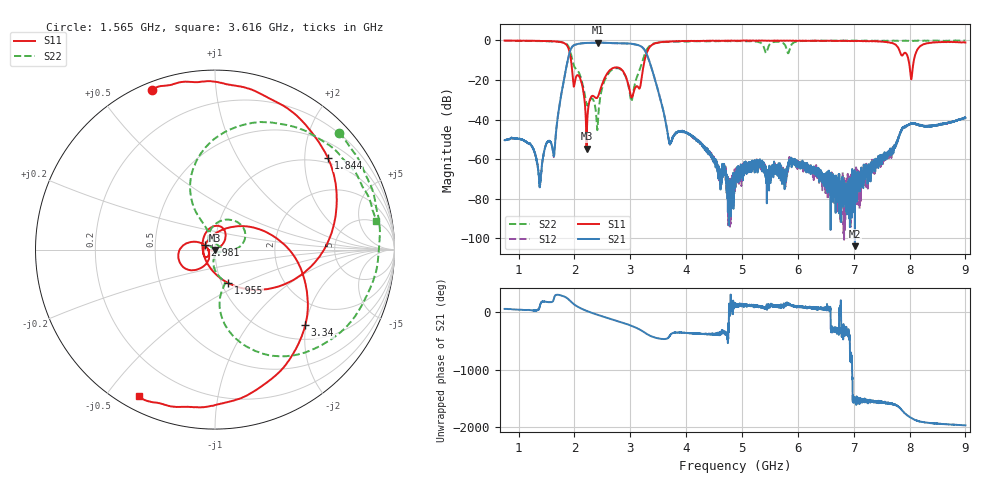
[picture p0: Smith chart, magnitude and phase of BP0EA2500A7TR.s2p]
!Agilent Technologies,E8358A,US41080443,A.07.50.56
!Agilent E8358A: A.07.50.56
!Date: Friday, November 20, 2015 10:47:14
!Correction: S11(Full 2 Port(1,2))
!S21(Full 2 Port(1,2))
!S12(Full 2 Port(1,2))
!S22(Full 2 Port(1,2))
!S2P File: Measurements: S11, S21, S12, S22:
# Hz S  dB  R 50
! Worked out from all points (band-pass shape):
!   6401 points, 750 MHz to 9 GHz, reference 50 ohm
!   highest |S21| = -1.11 dB at 2.414 GHz (marker M1); lowest = -104.0 dB at 7.021 GHz (marker M2)
!   |S21| within 3 dB of the highest: 1.94 GHz to 3.238 GHz (1.298 GHz wide, 50.1 % of centre)
!   lowest |S11| = -54.8 dB at 2.217 GHz (marker M3), VSWR 1.00, Z = 50 - j0.176 ohm
!   |S11| at or under -10 dB: 1.939 GHz to 3.257 GHz (1.319 GHz wide, 50.8 % of centre); 7.983 GHz to 8.077 GHz (94.32 MHz wide, 1.17 % of centre)
!   |S22| runs from -45.3 to 0.0 dB; largest |S21 - S12| = 0.0055
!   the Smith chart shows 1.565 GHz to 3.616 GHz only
!   S11 on the Smith chart (normalised r, x): 1.565 GHz: 0.03, +0.68; 1.844 GHz: 0.86, +2.56; 1.955 GHz: 1.07, -0.42; 2.981 GHz: 0.89, +0.04; 3.34 GHz: 1.34, -1.98; 3.616 GHz: 0.06, -0.61
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7.5e8  -0.05 161.1  -50.34 53.8  -50.43 54.1  -0.18 131.6
1.211484e9  -0.16 141.1  -52.47 32.4  -52.49 32.3  -0.30 90.8
1.377773e9  -0.23 129.8  -74.27 98.5  -71.71 86.6  -0.35 71.2
1.564688e9  -0.38 111.5  -51.08 170.0  -51.16 169.5  -0.44 43.3
1.64332e9  -0.46 99.7  -56.13 -92.6  -55.97 -93.4  -0.54 28.4
1.844414e9  -1.83 39.1  -14.98 -104.5  -15.02 -104.6  -1.44 -30.9
1.955273e9  -13.99 -68.5  -3.37 164.8  -3.40 164.8  -8.99 -85.0
2.12543e9  -21.07 48.6  -1.46 58.3  -1.50 58.3  -19.68 -92.1
2.216953e9  -54.76 -74.8  -1.25 19.6  -1.28 19.6  -32.11 -70.8
2.41418e9  -28.70 -148.7  -1.11 -48.8  -1.14 -48.8  -44.56 -152.6
2.665547e9  -14.32 -145.5  -1.31 -125.1  -1.34 -125.0  -14.96 69.1
2.981367e9  -24.19 157.0  -1.58 135.7  -1.61 135.7  -24.98 2.0
3.206953e9  -18.30 67.7  -3.24 34.6  -3.26 34.6  -11.55 116.6
3.339727e9  -3.66 -40.0  -10.31 -45.8  -10.37 -45.4  -2.90 76.7
3.500859e9  -1.06 -96.8  -25.56 -98.8  -25.63 -98.4  -1.04 31.0
3.615586e9  -0.70 -117.5  -38.59 -109.5  -38.68 -109.8  -0.78 10.2
4.875e9  -0.12 173.6  -67.93 108.3  -72.50 95.8  -0.30 -107.5
6.25043e9  -0.10 171.2  -65.26 73.0  -65.32 70.6  -0.20 -169.0
7.021289e9  -0.21 153.7  -103.99 -129.1  -72.10 -50.2  -0.18 170.7
7.625859e9  -0.95 118.2  -57.43 -135.7  -57.57 -131.9  -0.17 155.2
8.091211e9  -8.21 -142.7  -42.03 -73.1  -42.05 -72.9  -0.13 142.4
9e9  -1.02 90.0  -39.05 -169.1  -38.99 -170.7  -0.07 118.4
